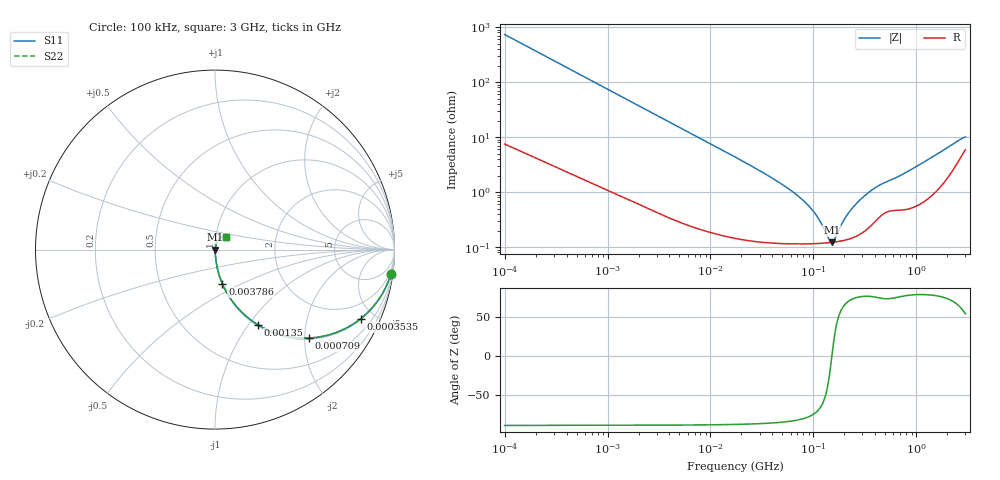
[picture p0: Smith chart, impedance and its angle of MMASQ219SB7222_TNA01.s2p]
! MMASQ219SB7222_TNA01  S-PARAMETER MODEL  ( Standard Model )
! Model Generated by TAIYO YUDEN Corporation (http://www.ty-top.com)
! Version 1.0
! TAIYO YUDEN Control No. 220601
! Copyright(c) 2013 TAIYO YUDEN CO.,LTD. All Rights Reserved.
! Product Description (link to TY-COMPAS)
! https://ds.yuden.co.jp/TYCOMPAS/or/detail?pn=MMASQ219SB7222KTNA01&u=M
! Products Name : Multilayer Ceramic Capacitors
! Characteristics :
!  Capacitance : 2200 [pF] , Rated Voltage : 250 [V] , TCC : X7R
!  Case Size : 2.0 x 1.25 / 0.079 x 0.049 [mm/inch] , Thickness : 0.85 / 0.033 [mm/inch]
!  (Conditions: Temperature = 25 [degC] , DC Bias Voltage = 0 [V])
! External Node Assignments :
!  1  o---| |---o  2
! GND o---------o GND
! Frequency Range : 100kHz  -  3GHz  [ 401 STEP ]
# MHZ S RI R 50
! Freq[MHz].  S11 Real  S11 Imag  S21 Real  S21 Imag  S12 Real  S12 Imag  S22 Real  S22 Imag
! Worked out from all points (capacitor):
!   401 points, 100 kHz to 3 GHz, reference 50 ohm
!   read as one part in series: C = 2.17 nF near 105.3 kHz
!   lowest |Z| = 122 mohm at 150.9 MHz (marker M1)
!   series resonance near 151.3 MHz, so ESL is about 510 pH
!   S11 on the Smith chart (normalised r, x): 100 kHz: 1, -15; 353.5 kHz: 1.05, -4.19; 709 kHz: 1.03, -2.10; 1.35 MHz: 1.02, -1.11; 3.786 MHz: 1.01, -0.40; 3 GHz: 1.12, +0.16
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0.1  0.9804 -0.1335  0.0196 0.1335  0.0196 0.1335  0.9804 -0.1335
0.205778  0.9252 -0.2574  0.0748 0.2574  0.0748 0.2574  0.9252 -0.2574
0.353547  0.8112 -0.3852  0.1888 0.3852  0.1888 0.3852  0.8112 -0.3852
0.562235  0.6341 -0.4751  0.3659 0.4751  0.3659 0.4751  0.6341 -0.4751
0.709011  0.524 -0.4926  0.476 0.4926  0.476 0.4926  0.524 -0.4926
1.350433  0.2384 -0.4186  0.7616 0.4186  0.7616 0.4186  0.2384 -0.4186
1.987766  0.1289 -0.3272  0.8711 0.3272  0.8711 0.3272  0.1289 -0.3272
3.161081  0.0573 -0.224  0.9427 0.224  0.9427 0.224  0.0573 -0.224
3.78604  0.0414 -0.1906  0.9586 0.1906  0.9586 0.1906  0.0414 -0.1906
17.7727  0.00321 -0.0422  0.9968 0.0422  0.9968 0.0422  0.00321 -0.0422
55.23785  0.00129 -0.012  0.9987 0.012  0.9987 0.012  0.00129 -0.012
77.22239  0.0012 -0.00734  0.9988 0.00734  0.9988 0.00734  0.0012 -0.00734
97.38194  0.00117 -0.00462  0.9988 0.00462  0.9988 0.00462  0.00117 -0.00462
116.6348  0.00117 -0.00268  0.9988 0.00268  0.9988 0.00268  0.00117 -0.00268
143.341  0.0012 -0.00055  0.9988 0.00055  0.9988 0.00055  0.0012 -0.00055
150.9232  0.00122 -2.44e-05  0.9988 2.44e-05  0.9988 2.44e-05  0.00122 -2.44e-05
163.0551  0.00124 0.000767  0.9988 -0.000767  0.9988 -0.000767  0.00124 0.000767
210.9903  0.00137 0.00349  0.9986 -0.00349  0.9986 -0.00349  0.00137 0.00349
259.3015  0.0016 0.00586  0.9984 -0.00586  0.9984 -0.00586  0.0016 0.00586
381.6779  0.0028 0.011  0.9972 -0.011  0.9972 -0.011  0.0028 0.011
547.5153  0.00471 0.0154  0.9953 -0.0154  0.9953 -0.0154  0.00471 0.0154
3000  0.0613 0.0727  0.9387 -0.0727  0.9387 -0.0727  0.0613 0.0727
